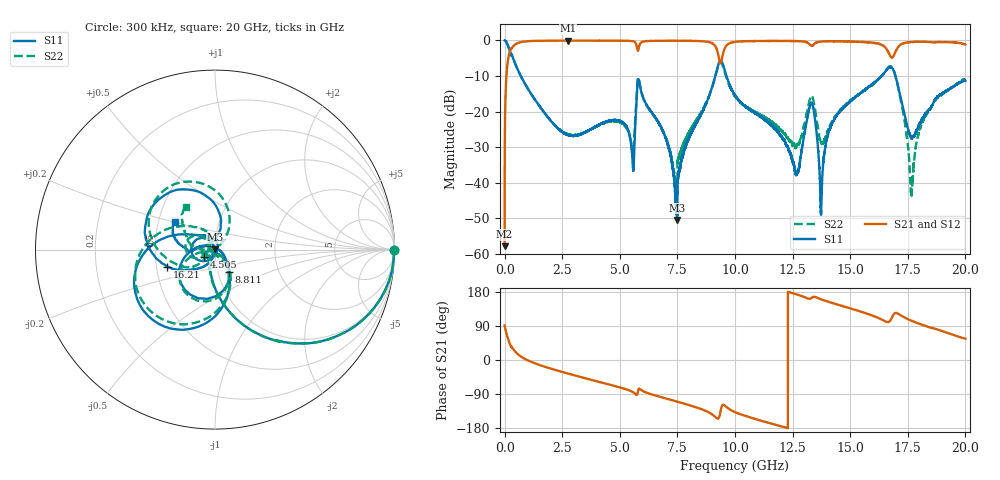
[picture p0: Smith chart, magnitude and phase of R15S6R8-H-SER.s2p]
!{R15S6R8}
!Johanson Technology Inc.
!www.johansontechnology.com
!Test Board Conditions:
!Substrate Type  RO4350B
!Substrate Thickness  20 mil
!Substrate Dk  3.66
!TL Type: GCPW
!TL Trace Width  34 mil
!TL Gap  10 mil
!Electrode orientation  Horizontal
!DUT TOPOLOGY	SERIES
!Mounting Pad LxW  26x52 mil
! Created Sat Feb  6 14:00:55 2021
# hz S ma R 50
! 2 Port Network Data from SP1.SP block
! freq  magS11  angS11  magS21  angS21  magS12  angS12  magS22  angS22
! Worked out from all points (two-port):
!   20001 points, 300 kHz to 20 GHz, reference 50 ohm
!   highest |S21| = -0.03 dB at 2.753 GHz (marker M1); lowest = -57.8 dB at 300 kHz (marker M2)
!   |S21| within 3 dB of the highest: 235 MHz to 9.235 GHz (9 GHz wide, 190 % of centre); 9.509 GHz to 16.64 GHz (7.126 GHz wide, 54.5 % of centre)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
!   lowest |S11| = -50.5 dB at 7.487 GHz (marker M3), VSWR 1.01, Z = 50.2 + j0.207 ohm
!   |S11| at or under -10 dB: 704.9 MHz to 9.143 GHz (8.438 GHz wide, 171 % of centre); 9.631 GHz to 16.36 GHz (6.733 GHz wide, 51.8 % of centre); 16.97 GHz to end of sweep
!   |S22| runs from -43.7 to 0.0 dB; largest |S21 - S12| = 0.015
!   S11 on the Smith chart (normalised r, x): 300 kHz: open; 4.505 GHz: 0.88, -0.08; 8.811 GHz: 1.13, -0.28; 16.21 GHz: 0.57, -0.12; 20 GHz: 0.61, +0.20
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300000  1 -0.3  0.001284 91.0  0.001318 88.9  0.9976 -0.2
1.093e8  0.9039 -26.6  0.4219 63.2  0.423 63.1  0.9047 -26.5
2.823e8  0.6318 -54.2  0.7668 35.2  0.7674 35.2  0.6321 -54.2
2.7533e9  0.04697 -116.8  0.9968 -35.9  0.9958 -35.8  0.04781 -133.3
3.3343e9  0.04856 -122.2  0.9956 -45.4  0.9951 -45.5  0.04913 -147.3
4.5053e9  0.07389 -144.5  0.9926 -64.2  0.9914 -64.2  0.07208 -162.4
5.5563e9  0.01946 -145.6  0.978 -84.0  0.9785 -84.0  0.02758 -117.1
5.8353e9  0.2696 -133.7  0.8199 -75.5  0.8205 -75.5  0.2789 -131.9
6.6673e9  0.07134 162.1  0.9885 -95.8  0.9892 -95.8  0.07134 -169.9
7.4873e9  0.002991 43.4  0.9904 -109.8  0.991 -109.8  0.00706 -103.1
8.8113e9  0.1459 -57.4  0.9584 -136.6  0.9589 -136.6  0.1496 -55.4
9.3703e9  0.5247 -134.4  0.48 -136.5  0.4837 -136.5  0.4983 -140.1
1.00003e10  0.1696 150.1  0.955 -137.6  0.9563 -137.6  0.1638 130.2
1.26743e10  0.01362 -10.8  0.9796 173.2  0.9813 173.1  0.03296 168.9
1.33343e10  0.1312 172.2  0.8397 164.2  0.8402 164.2  0.1664 167.6
1.37443e10  0.004125 -141.2  0.9684 160.0  0.9674 160.1  0.03678 165.5
1.42803e10  0.07412 -113.2  0.9764 149.4  0.9746 149.5  0.07811 -137.6
1.62063e10  0.2815 -160.5  0.9024 111.3  0.9005 111.3  0.2795 -171.1
1.66673e10  0.4117 159.8  0.6758 100.2  0.6627 100.6  0.4231 147.7
1.76633e10  0.04293 118.6  0.9543 103.5  0.9497 103.7  0.007371 113.4
1.82163e10  0.08767 172.7  0.9587 91.2  0.9591 90.8  0.08072 177.8
2e10  0.2711 145.2  0.877 56.3  0.8693 56.1  0.2877 123.6
